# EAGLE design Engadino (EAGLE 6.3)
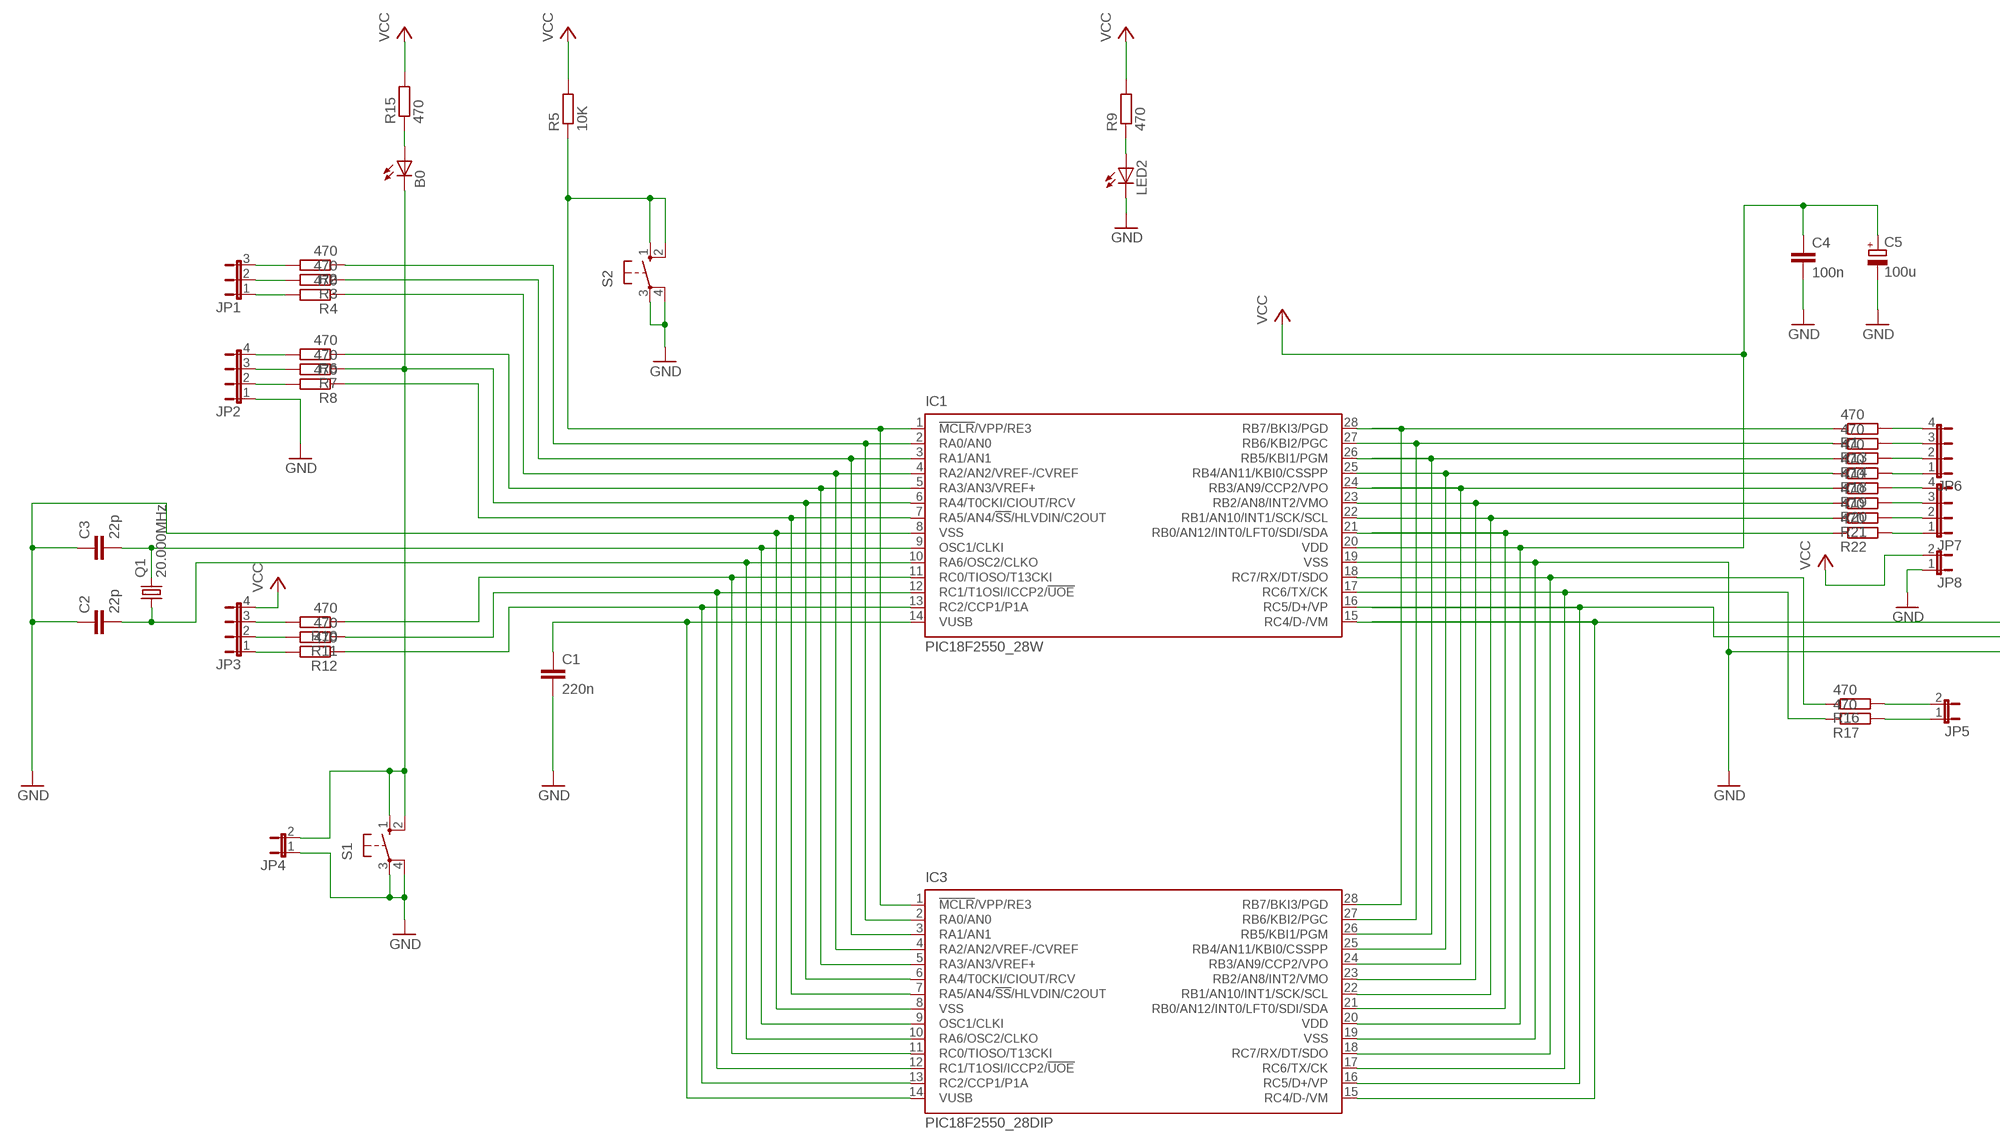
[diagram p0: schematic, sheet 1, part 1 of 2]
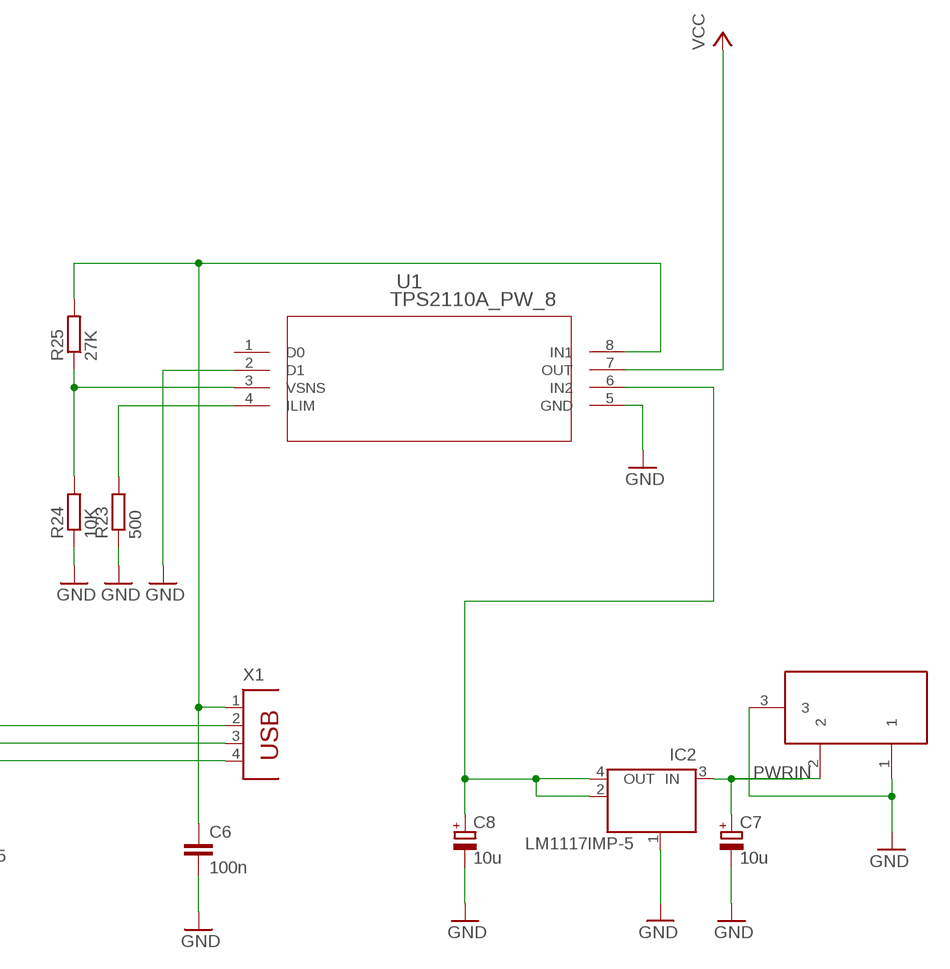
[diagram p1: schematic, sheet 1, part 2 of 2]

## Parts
B0  LEDCHIPLED_0805  [CHIPLED_0805]
C1  220n  C-EUC2012  [C2012]
C2  22p  C-EUC2012  [C2012]
C3  22p  C-EUC2012  [C2012]
C4  100n  C-EUC2012  [C2012]
C5  100u  CPOL-EU085CS-1AR  [085CS_1AR]
C6  100n  C-EUC2012  [C2012]
C7  10u  CPOL-EU085CS-1AR  [085CS_1AR]
C8  10u  CPOL-EU085CS-1AR  [085CS_1AR]
IC1  PIC18F2550_28W  [SO28W]
IC2  LM1117IMP-5  MC33269ST-3.3T3  [SOT223]
IC3  PIC18F2550_28DIP  [DIL28-3]
JP1  JP2E  [JP2]
JP2  JP4E  [JP4]
JP3  JP4E  [JP4]
JP4  JP1E  [JP1]
JP5  JP1E  [JP1]
JP6  JP4E  [JP4]
JP7  JP4E  [JP4]
JP8  JP1E  [JP1]
LED2  LEDCHIPLED_0805  [CHIPLED_0805]
Q1  20.000MHz  CRYSTALHC49S  [HC49/S]
R1  470  R-EU_R2012  [R2012]
R2  470  R-EU_R2012  [R2012]
R3  470  R-EU_R2012  [R2012]
R4  470  R-EU_R2012  [R2012]
R5  10K  R-EU_R2012  [R2012]
R6  470  R-EU_R2012  [R2012]
R7  470  R-EU_R2012  [R2012]
R8  470  R-EU_R2012  [R2012]
R9  470  R-EU_R2012  [R2012]
R10  470  R-EU_R2012  [R2012]
R11  470  R-EU_R2012  [R2012]
R12  470  R-EU_R2012  [R2012]
R13  470  R-EU_R2012  [R2012]
R14  470  R-EU_R2012  [R2012]
R15  470  R-EU_R2012  [R2012]
R16  470  R-EU_R2012  [R2012]
R17  470  R-EU_R2012  [R2012]
R18  470  R-EU_R2012  [R2012]
R19  470  R-EU_R2012  [R2012]
R20  470  R-EU_R2012  [R2012]
R21  470  R-EU_R2012  [R2012]
R22  470  R-EU_R2012  [R2012]
R23  500  R-EU_R2012  [R2012]
R24  10K  R-EU_R2012  [R2012]
R25  27K  R-EU_R2012  [R2012]
S1  10-XX  [B3F-10XX]
S2  10-XX  [B3F-10XX]
U1  TPS2110A_PW_8  [PW8]
X1  PN61729  [PN61729]
X2  DC21MMX  [DC-21MM]

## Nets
+5V: C8.+ IC2.2(OUT) IC2.4(OUT) U1.6(IN2)
GND: C1.2 C2.1 C3.1 C4.2 C5.- C6.2 C7.- C8.- IC1.8(VSS) IC1.19(VSS) IC2.1(GND/ADJ) IC3.8(VSS) IC3.19(VSS) JP2.1 JP4.1 JP8.1 LED2.C R23.1 R24.1 S1.3(P) S1.4(P1) S2.3(P) S2.4(P1) U1.2(D1) U1.5(GND) X1.4 X2.1 X2.3
GND2: IC1.21(RB0/AN12/INT0/LFT0/SDI/SDA) IC3.21(RB0/AN12/INT0/LFT0/SDI/SDA) R22.1
N$1: JP1.3 R2.2
N$2: IC1.15(RC4/D-/VM) IC3.15(RC4/D-/VM) X1.2
N$3: JP5.2 R16.2
N$4: JP5.1 R17.2
N$5: JP6.1 R18.2
N$9: JP1.2 R3.2
N$10: IC1.25(RB4/AN11/KBI0/CSSPP) IC3.25(RB4/AN11/KBI0/CSSPP) R18.1
N$11: JP7.4 R19.2
N$12: JP7.3 R20.2
N$13: JP6.4 R1.2
N$14: JP7.2 R21.2
N$15: IC1.24(RB3/AN9/CCP2/VPO) IC3.24(RB3/AN9/CCP2/VPO) R19.1
N$16: IC1.23(RB2/AN8/INT2/VMO) IC3.23(RB2/AN8/INT2/VMO) R20.1
N$17: JP1.1 R4.2
N$19: JP2.4 R6.2
N$20: JP2.3 R7.2
N$21: JP2.2 R8.2
N$23: JP3.3 R10.2
N$24: JP3.2 R11.2
N$25: JP3.1 R12.2
N$27: IC1.3(RA1/AN1) IC3.3(RA1/AN1) R3.1
N$33: JP6.3 R13.2
N$34: JP6.2 R14.2
N$35: LED2.A R9.1
N$38: IC1.22(RB1/AN10/INT1/SCK/SCL) IC3.22(RB1/AN10/INT1/SCK/SCL) R21.1
N$39: JP7.1 R22.2
N$41: IC1.18(RC7/RX/DT/SDO) IC3.18(RC7/RX/DT/SDO) R16.1
N$42: B0.A R15.1
N$43: IC1.28(RB7/BKI3/PGD) IC3.28(RB7/BKI3/PGD) R1.1
N$44: IC1.27(RB6/KBI2/PGC) IC3.27(RB6/KBI2/PGC) R13.1
N$45: IC1.17(RC6/TX/CK) IC3.17(RC6/TX/CK) R17.1
N$46: R23.2 U1.4(ILIM)
N$47: R24.2 R25.1 U1.3(VSNS)
N$48: IC1.26(RB5/KBI1/PGM) IC3.26(RB5/KBI1/PGM) R14.1
N$49: C6.1 R25.2 U1.8(IN1) X1.1
N$51: C1.1 IC1.14(VUSB) IC3.14(VUSB)
N$52: C3.2 IC1.9(OSC1/CLKI) IC3.9(OSC1/CLKI) Q1.2
N$53: C2.2 IC1.10(RA6/OSC2/CLKO) IC3.10(RA6/OSC2/CLKO) Q1.1
N$54: IC1.16(RC5/D+/VP) IC3.16(RC5/D+/VP) X1.3
N$55: IC1.2(RA0/AN0) IC3.2(RA0/AN0) R2.1
N$57: IC1.4(RA2/AN2/VREF-/CVREF) IC3.4(RA2/AN2/VREF-/CVREF) R4.1
N$58: IC1.5(RA3/AN3/VREF+) IC3.5(RA3/AN3/VREF+) R6.1
N$59: B0.C IC1.6(RA4/T0CKI/CIOUT/RCV) IC3.6(RA4/T0CKI/CIOUT/RCV) JP4.2 R7.1 S1.1(S) S1.2(S1)
N$60: IC1.7(RA5/AN4/!SS!/HLVDIN/C2OUT) IC3.7(RA5/AN4/!SS!/HLVDIN/C2OUT) R8.1
N$61: IC1.11(RC0/TIOSO/T13CKI) IC3.11(RC0/TIOSO/T13CKI) R10.1
N$62: IC1.12(RC1/T1OSI/ICCP2/!UOE) IC3.12(RC1/T1OSI/ICCP2/!UOE) R11.1
N$63: IC1.13(RC2/CCP1/P1A) IC3.13(RC2/CCP1/P1A) R12.1
N$64: IC1.1(!MCLR!/VPP/RE3) IC3.1(!MCLR!/VPP/RE3) R5.1 S2.1(S) S2.2(S1)
PWRIN: C7.+ IC2.3(IN) X2.2
VCC: C4.1 C5.+ IC1.20(VDD) IC3.20(VDD) JP3.4 JP8.2 R5.2 R9.2 R15.2 U1.7(OUT)
Unconnected: U1.1(D0)

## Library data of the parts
B0 LED2 = led:LED: LED
C1-C4 C6 = rcl:C-EU: CAPACITOR, European symbol
C5 C7 C8 = rcl:CPOL-EU: POLARIZED CAPACITOR, European symbol
IC1 IC3 = microchip:PIC18F2*_28: USB Microcontrollers with nanoWatt Technology High-Performance, Enhanced Flash, 28/40/44-Pin, Source: http://ww1.microchip.com/downloads/en/devicedoc/39632c.pdf
IC2 = linear:MC33269ST*: Adjustable Output Low Dropout Voltage Regulator 800 mA Source: http://www.onsemi.com/pub/Collateral/MC33269-D.PDF
JP1 = jumper:JP2E: JUMPER
JP2 JP3 JP6 JP7 = jumper:JP4E: JUMPER
JP4 JP5 JP8 = jumper:JP1E: JUMPER
Q1 = crystal:CRYSTAL: CRYSTAL
R1-R25 = rcl:R-EU_: RESISTOR, European symbol
S1 S2 = switch-omron:10-XX: OMRON SWITCH; MPN: B3F-1000; OC_FARNELL: 176432; OC_NEWARK: 36M3542
U1 = TPS2110A:TPS2110A_PW_8; DATASHEETURL: http://www.ti.com/lit/gpn/TPS2110A; DESCRIPTION: Autoswitching Power Mux; FAMILY_NAME: POWER MULTIPLEXER (MUX); GENERIC_PART_NUMBER: TPS2110A; INDUSTRY_STD_PKG_TYPE: TSSOP; MANUFACTURER: Texas Instruments; MANUFACTURER_PART_NUMBER: tps2110a_pw_8; PACKAGE_DESIGNATOR: PW; PIN_COUNT: 8; VENDOR: Texas Instruments
X1 = con-berg:PN61729: BERG USB connector
X2 = powersupply:DC21MM

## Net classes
0 default: width 0.203 mm, drill 0.406 mm, clearance 0.203 mm
2 gnd: width 0.305 mm, drill 0.711 mm, clearance 0.203 mm

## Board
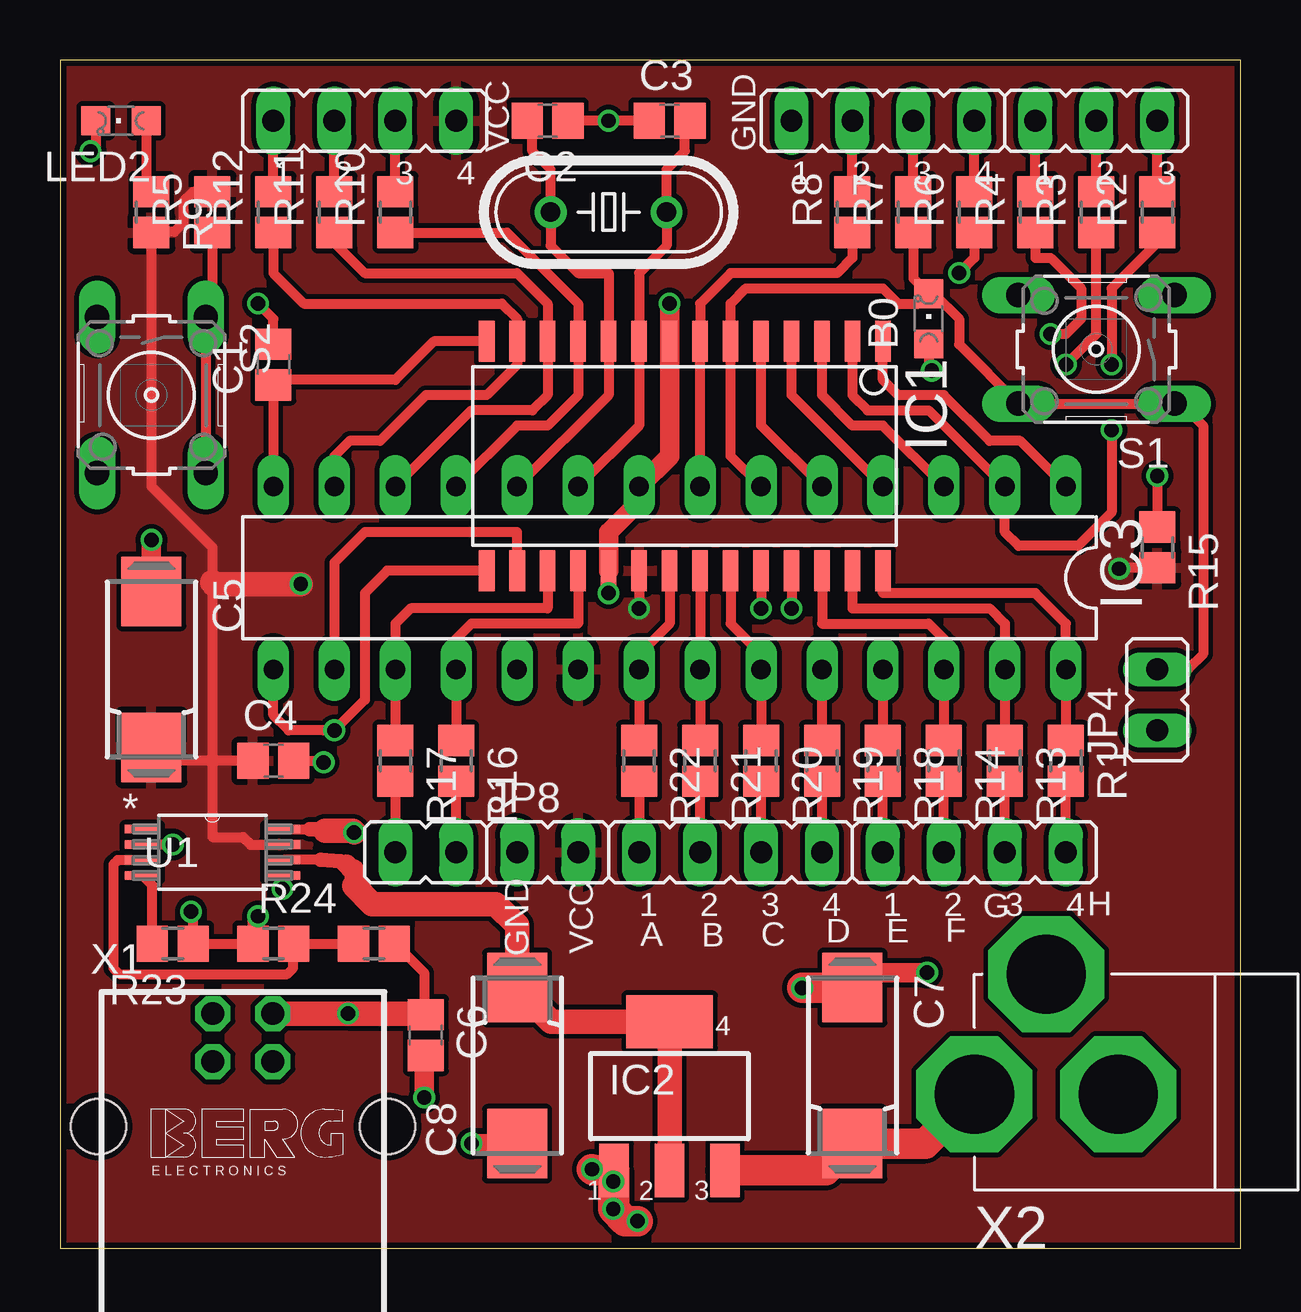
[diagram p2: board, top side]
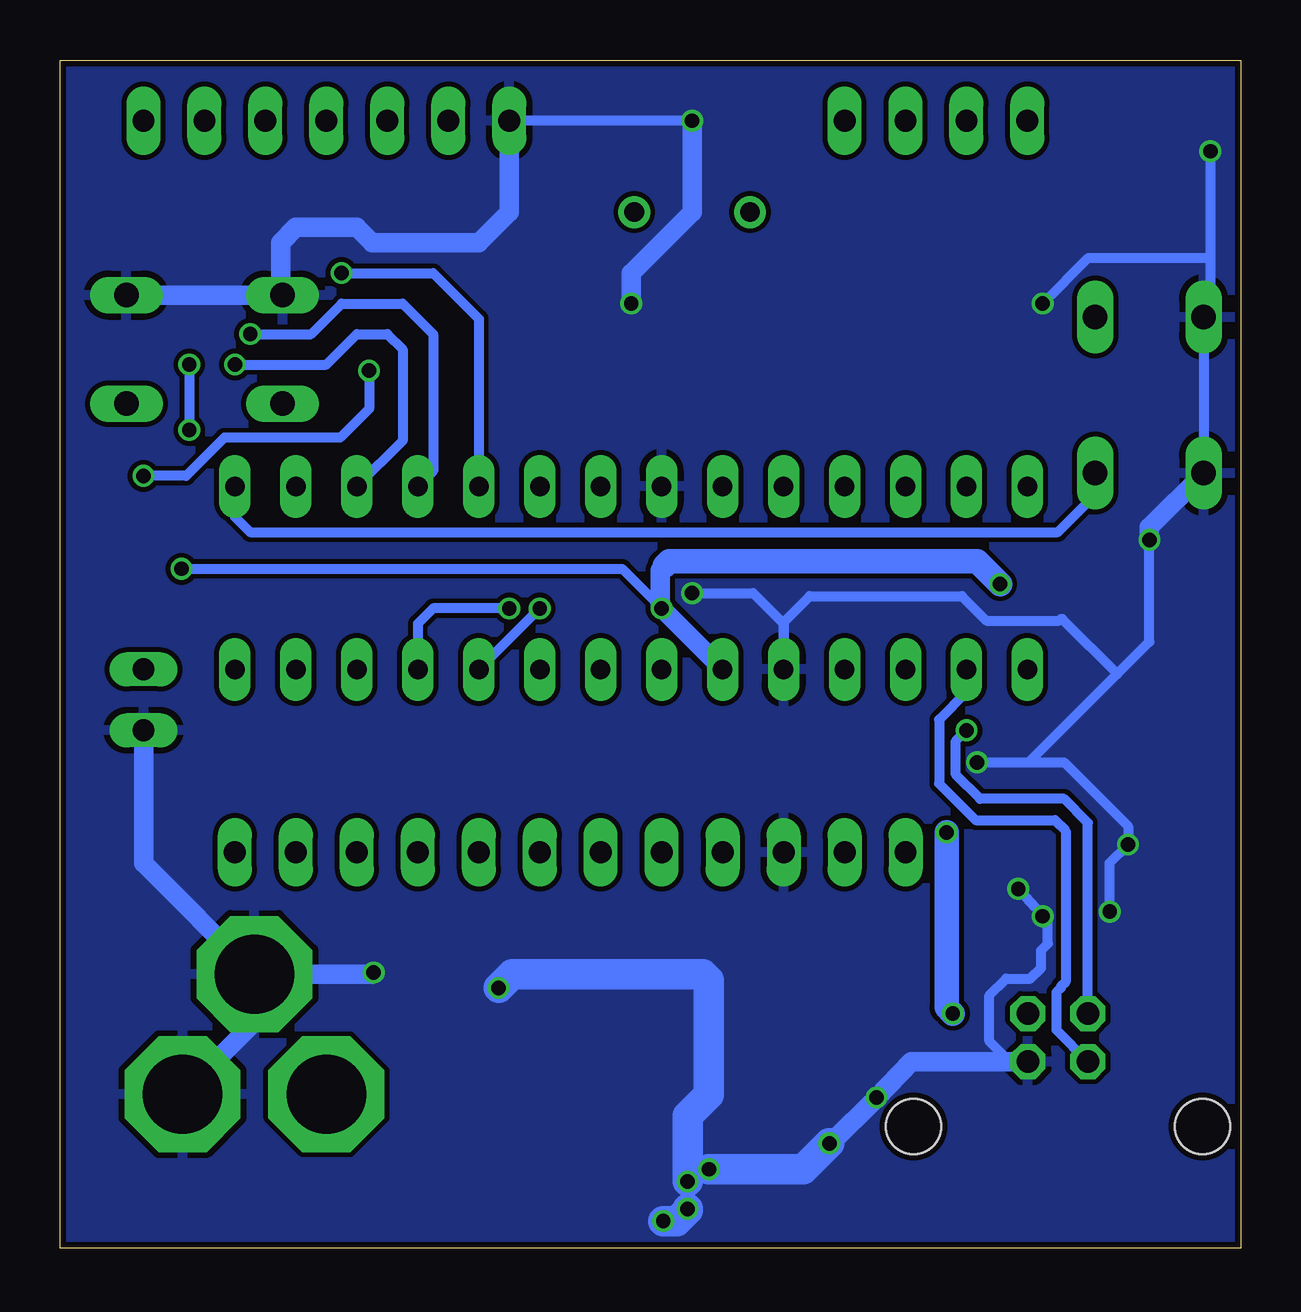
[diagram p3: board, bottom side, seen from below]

Size 49.2 x 49.52 mm. Coordinates in mm from the lower left corner, seen from the top.
Outline: 0,0 49.2,0 49.2,49.52 0,49.52 0,0
Copper layers (1*16): Top 0.035mm / dielectric 1.5mm / Bottom 0.035mm
Design rules "ITead_rule": minimum track width 6mil, minimum drill 12mil, track to track 6mil, track to pad 6mil, pad to pad 6mil, via to via 6mil, smd to smd 0mil, copper to edge 10mil, drill to drill 10mil, minimum pad ring 10mil, minimum via ring 6mil, stop-mask expansion 2mil, vias tented up to drill 100mil, thermal gap 10mil

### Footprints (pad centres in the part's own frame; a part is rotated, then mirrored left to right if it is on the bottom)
CHIPLED_0805 = smd 1.2 x 1.2: A 0,-1.05; C 0,1.05
C2012 = smd 1.3 x 1.5: 1 -0.85,0; 2 0.85,0
085CS_1AR = smd 2.9 x 2.5: + 3.25,0; - -3.25,0
SO28W = smd 0.65 x 1.7: 1 -7.62,-4.78; 2 -6.35,-4.78; 3 -5.08,-4.78; 4 -3.81,-4.78; 5 -2.54,-4.78; 6 -1.27,-4.78; 7 0,-4.78; 8 1.27,-4.78; 9 2.54,-4.78; 10 3.81,-4.78; 11 5.08,-4.78; 12 6.35,-4.78; 13 7.62,-4.78; 14 8.89,-4.78; 15 8.89,4.78; 16 7.62,4.78; 17 6.35,4.78; 18 5.08,4.78; 19 3.81,4.78; 20 2.54,4.78; 21 1.27,4.78; 22 0,4.78; 23 -1.27,4.78; 24 -2.54,4.78; 25 -3.81,4.78; 26 -5.08,4.78; 27 -6.35,4.78; 28 -7.62,4.78
SOT223 = smd 1.219 x 2.235: 1 -2.311,-3.099; 2 0,-3.099; 3 2.311,-3.099 | smd 3.6 x 2.2: 4 0,3.099
DIL28-3 = drill 0.813 long: 1 -16.51,-3.81; 2 -13.97,-3.81; 3 -11.43,-3.81; 4 -8.89,-3.81; 5 -6.35,-3.81; 6 -3.81,-3.81; 7 -1.27,-3.81; 8 1.27,-3.81; 9 3.81,-3.81; 10 6.35,-3.81; 11 8.89,-3.81; 12 11.43,-3.81; 13 13.97,-3.81; 14 16.51,-3.81; 15 16.51,3.81; 16 13.97,3.81; 17 11.43,3.81; 18 8.89,3.81; 19 6.35,3.81; 20 3.81,3.81; 21 1.27,3.81; 22 -1.27,3.81; 23 -3.81,3.81; 24 -6.35,3.81; 25 -8.89,3.81; 26 -11.43,3.81; 27 -13.97,3.81; 28 -16.51,3.81
JP2 = drill 0.914 long: 1 -2.54,0; 2 0,0; 3 2.54,0
JP4 = drill 0.914 long: 1 -3.81,0; 2 -1.27,0; 3 1.27,0; 4 3.81,0
JP1 = drill 0.914 long: 1 0,-1.27; 2 0,1.27
HC49/S = drill 0.813: 1 -2.413,0; 2 2.413,0
R2012 = smd 1.3 x 1.5: 1 -0.85,0; 2 0.85,0
B3F-10XX = drill 1.016 long: 1 -3.251,2.261; 2 3.251,2.261; 3 -3.251,-2.261; 4 3.251,-2.261
PW8 = smd 1.473 x 0.356: 1 -2.921,0.965; 2 -2.921,0.33; 3 -2.921,-0.33; 4 -2.921,-0.965; 5 2.921,-0.965; 6 2.921,-0.33; 7 2.921,0.33; 8 2.921,0.965
PN61729 = drill 0.95 octagon: 1 1.25,4.71; 2 -1.25,4.71; 3 -1.25,2.71; 4 1.25,2.71 | hole 2.3: -6.02,0; 6.02,0
DC-21MM = drill 3.302 pad 4.826 octagon: 1 -5.08,-3.353; 2 -0.076,-6.35; 3 -0.076,-0.356

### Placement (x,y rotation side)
B0  36.2,38.73 0 top
C1  8.89,36.83 90 top
C2  20.32,46.99 180 top
C3  25.4,46.99 0 top
C4  8.89,20.32 0 top
C5  3.81,24.13 270 top
C6  15.24,8.89 270 top
C7  33.02,7.62 270 top
C8  19.05,7.62 90 top
IC1  26.67,33.02 180 top
IC2  25.4,6.35 0 top
IC3  25.4,27.94 180 top
JP1  43.18,46.99 0 top
JP2  34.29,46.99 0 top
JP3  12.7,46.99 0 top
JP4  45.72,22.86 0 top
JP5  15.24,16.51 270 top
JP6  38.1,16.51 0 top
JP7  27.94,16.51 0 top
JP8  20.32,16.51 270 top
LED2  2.54,46.99 90 top
Q1  22.86,43.18 0 top
R1  41.91,20.32 270 top
R2  45.72,43.18 90 top
R3  43.18,43.18 90 top
R4  40.64,43.18 90 top
R5  6.35,43.18 90 top
R6  38.1,43.18 90 top
R7  35.56,43.18 90 top
R8  33.02,43.18 90 top
R9  3.81,43.18 270 top
R10  13.97,43.18 90 top
R11  11.43,43.18 90 top
R12  8.89,43.18 90 top
R13  39.37,20.32 270 top
R14  36.83,20.32 270 top
R15  45.72,29.21 270 top
R16  16.51,20.32 270 top
R17  13.97,20.32 270 top
R18  34.29,20.32 270 top
R19  31.75,20.32 270 top
R20  29.21,20.32 270 top
R21  26.67,20.32 270 top
R22  24.13,20.32 270 top
R23  4.7,12.7 180 top
R24  8.89,12.7 0 top
R25  13.08,12.7 0 top
S1  43.18,37.47 180 top
S2  3.81,35.56 270 top
U1  6.35,16.51 0 top
X1  7.62,5.08 0 top
X2  44.45,6.35 270 top

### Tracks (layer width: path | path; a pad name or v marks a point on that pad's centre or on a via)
+5V
  Top 0.406: 10.86,16.19 9.32,16.19 U1.6
  Top 0.61: 11.94,16 11.81,16 11.68,16.13 10.86,16.19
  Top 0.813: 12.26,15.11 12.26,15.81 12.13,15.81 11.94,16
  Top 1.016: IC2.2 IC2.4 20.47,9.45 C8.+ 19.05,13.46 18.16,14.35 13.02,14.35 12.26,15.11
GND  (via drill 0.6)
  Top 0.406: IC1.19 v22.86,27.3 | LED2.C 1.49,45.94 v1.27,45.72 | C1.2 8.89,38.73 v8.26,39.37 | C2.1 v22.86,46.99 C3.1 | C4.2 10.92,20.32 v10.99,20.26 | v8.26,13.84 8.04,13.82 R24.1 R23.1 5.55,13.82 v5.46,14.03 | v9.27,14.99 U1.5 | v4.7,16.83 3.44,16.83 U1.2
  Top 0.813: IC1.19 22.86,29.84 24.13,31.11 IC3.8 25.4,33.02 IC1.8 v25.4,39.37 | C5.- v3.81,29.53 | v36.13,11.49 33.64,11.49 C7.- | C8.- 17.16,4.37 v17.14,4.38 | v15.18,6.29 15.18,7.98 C6.2
  Top 1.27: v22.16,3.3 22.21,3.25 IC2.1 23.09,1.69 v23.05,1.65 | v24.07,1.14 23.56,1.14 v23.05,1.65 | v23.05,1.65 v23.05,2.79 | v30.92,10.86 33.01,10.86 C7.-
  Bottom 0.406: v22.86,27.3 20.32,27.3 19.05,26.04 IC3.19 19.05,26.1 17.97,27.18 11.62,27.18 10.6,26.16 7.56,26.16 7.49,26.23 7.43,26.23 5.14,23.94 | v1.27,45.72 1.27,41.27 | 1.27,41.27 1.27,39.09 S2.3 S2.4 | v8.26,39.37 6.35,41.27 1.27,41.27 | v22.86,46.99 JP2.1 | v10.99,20.26 8.83,20.26 | 8.83,20.26 5.14,23.94 | 5.14,23.94 3.81,25.27 v3.81,29.53 | v9.27,14.99 v8.26,13.84 8.04,13.82 R24.1 8.32,12.42 8.32,11.68 8.76,11.24 9.78,11.24 10.48,10.54 10.48,8.64 9.63,7.79 X1.4 | v5.46,14.03 5.46,16.07 v4.7,16.83 4.7,17.59 7.37,20.26 8.83,20.26
  Bottom 0.813: v25.4,39.37 25.4,40.64 22.86,43.18 v22.86,46.99 | JP2.1 30.48,43.18 31.75,41.91 36.2,41.91 36.83,42.55 39.37,42.55 40.01,41.91 40.01,39.8 S1.4 S1.3 | v3.81,29.53 3.81,30.05 S2.4 | JP4.1 45.72,16.05 X2.1 | X2.1 41.1,9.42 X2.3 | X2.1 36.2,11.43 v36.13,11.49 | v17.14,4.38 17.08,4.38 v15.18,6.29 13.74,7.79 X1.4
  Bottom 1.27: v22.16,3.3 18.22,3.3 v17.14,4.38 | v23.05,1.65 23.05,1.59 23.5,1.14 v24.07,1.14 | v23.05,2.79 23.05,5.52 22.16,6.41 22.16,11.18 22.42,11.43 30.35,11.43 v30.92,10.86
  pour Bottom: -1.27,49.53 49.53,49.53 49.53,-1.27 -1.27,-1.27
GND2
  Top 0.406: IC1.21 25.4,26.04 24.13,24.77 IC3.21 R22.1
N$1
  Top 0.406: R2.2 JP1.3
N$2  (via drill 0.6)
  Top 0.406: IC1.15 13.63,28.24 12.7,27.3 12.7,22.86 v11.43,21.59 10.99,21.59 9.53,21.59 8.89,22.23 IC3.15
  Bottom 0.406: X1.2 6.37,17.74 7.37,18.73 10.86,18.73 11.87,19.75 11.87,21.14 v11.43,21.59
N$3
  Top 0.406: JP5.2 R16.2
N$4
  Top 0.406: R17.2 JP5.1
N$5
  Top 0.406: JP6.1 R18.2
N$9
  Top 0.406: R3.2 JP1.2
N$10  (via drill 0.6)
  Top 0.406: IC1.25 v30.48,26.67 | IC3.25 R18.1
  Bottom 0.406: v30.48,26.67 33.66,26.67 34.29,26.04 IC3.25
N$11
  Top 0.406: JP7.4 R19.2
N$12
  Top 0.406: JP7.3 R20.2
N$13
  Top 0.406: JP6.4 R1.2
N$14
  Top 0.406: JP7.2 R21.2
N$15  (via drill 0.6)
  Top 0.406: IC1.24 v29.21,26.67 | R19.1 IC3.24
  Bottom 0.406: v29.21,26.67 IC3.24
N$16
  Top 0.406: IC1.23 27.94,26.04 29.21,24.77 IC3.23 R20.1
N$17
  Top 0.406: R4.2 JP1.1
N$19
  Top 0.406: R6.2 JP2.4
N$20
  Top 0.406: R7.2 JP2.3
N$21
  Top 0.406: R8.2 JP2.2
N$23
  Top 0.406: R10.2 JP3.3
N$24
  Top 0.406: R11.2 JP3.2
N$25
  Top 0.406: R12.2 JP3.1
N$27  (via drill 0.6)
  Top 0.406: IC3.3 34.29,34.29 33.02,34.29 31.75,35.56 IC1.3 | v41.91,36.83 43.18,38.1 R3.1
  Bottom 0.406: v41.91,36.83 38.1,36.83 36.83,38.1 35.56,38.1 34.92,37.47 34.92,33.66 IC3.3
N$33
  Top 0.406: JP6.3 R13.2
N$34
  Top 0.406: JP6.2 R14.2
N$35
  Top 0.406: LED2.A 3.59,44.25 R9.1
N$38
  Top 0.406: IC1.22 IC3.22 R21.1
N$39
  Top 0.406: R22.2 JP7.1
N$41
  Top 0.406: IC1.18 21.59,26.04 17.14,26.04 16.51,25.4 IC3.18 R16.1
N$42  (via drill 0.6)
  Top 0.406: B0.A 36.2,36.7 v36.32,36.58 | v45.72,32.19 R15.1
  Bottom 0.406: v36.32,36.58 36.32,34.99 37.53,33.78 42.35,33.78 43.94,32.19 v45.72,32.19
N$43
  Top 0.406: R1.1 IC3.28 41.91,26.04 40.64,27.3 34.29,27.3 IC1.28
N$44
  Top 0.406: IC1.27 33.02,26.67 38.73,26.67 39.37,26.04 IC3.27 R13.1
N$45
  Top 0.406: IC1.17 20.32,26.67 14.61,26.67 13.97,26.04 IC3.17 R17.1
N$46
  Top 0.406: R23.2 3.85,15.12 U1.4
N$47
  Top 0.406: R25.1 R24.2 9.72,12.68 9.72,11.68 9.46,11.43 2.48,11.43 2.22,11.68 2.22,16 2.4,16.18 U1.3
N$48
  Top 0.406: IC1.26 31.75,26.04 36.2,26.04 36.83,25.4 IC3.26 R14.1
N$49  (via drill 0.6)
  Top 0.406: R25.2 13.97,12.7 15.18,11.49 15.18,9.8 C6.1 | U1.8 10.4,17.48 10.41,17.46
  Top 0.61: 10.41,17.46 10.99,17.46 11.05,17.4
  Top 1.016: C6.1 15.24,9.79 v12,9.79 X1.1 | 11.05,17.4 12.19,17.4 v12.26,17.34
  Bottom 1.016: v12.26,17.34 12.26,10.04 v12,9.79
N$51
  Top 0.406: IC1.14 15.57,37.8 13.97,36.2 9.11,36.2 C1.1 IC3.14
N$52
  Top 0.406: IC3.9 24.13,34.29 IC1.9 24.13,40.64 25.27,41.78 Q1.2 25.27,44.96 26.04,45.72 26.04,46.77 C3.2
N$53
  Top 0.406: IC3.10 22.86,35.56 IC1.10 22.86,40.64 21.59,40.64 20.45,41.78 Q1.1 20.45,44.96 19.68,45.72 19.68,46.77 C2.2
N$54
  Top 0.406: IC1.16 19.05,29.84 12.7,29.84 11.43,28.57 IC3.16
  Bottom 0.406: IC3.16 11.43,23.18 12.57,22.04 12.57,19.37 11.05,17.84 7.75,17.84 7.3,17.4 7.3,11.11 7.49,10.92 7.49,10.86 7.68,10.67 7.68,9.1 X1.3
N$55  (via drill 0.6)
  Top 0.406: IC1.2 33.02,35.56 33.66,34.92 36.2,34.92 IC3.2 39.37,29.84 39.94,29.27 42.42,29.27 43.81,30.67 v43.81,34.1 | R2.1 45.72,41.91 43.81,40.01 v43.81,36.83
  Bottom 0.406: v43.81,36.83 v43.81,34.1
N$57  (via drill 0.6)
  Top 0.406: IC3.4 30.48,35.56 IC1.4 | R4.1 40.64,41.27 41.27,41.27 42.55,40.01 42.55,38.73 41.91,38.1 v41.27,38.1
  Bottom 0.406: v41.27,38.1 38.73,38.1 37.47,39.37 34.92,39.37 33.66,38.1 33.66,32.38 IC3.4
N$58  (via drill 0.6)
  Top 0.406: IC3.5 29.21,34.29 IC1.5 | R6.1 38.1,41.27 v37.47,40.64
  Bottom 0.406: v37.47,40.64 33.66,40.64 31.75,38.73 IC3.5
N$59
  Top 0.406: IC3.6 27.94,33.02 IC1.6 27.94,39.37 28.57,40.01 34.29,40.01 34.92,39.37 35.78,39.37 B0.C | R7.1 35.56,40.42 B0.C | B0.C 36.41,39.78 37.47,38.73 37.47,37.67 S1.2 S1.1 46.71,35.2 47.62,34.29 47.62,24.77 46.99,24.13 JP4.2
N$60
  Top 0.406: IC3.7 IC1.7 26.67,39.37 27.94,40.64 32.38,40.64 33.02,41.27 R8.1
N$61
  Top 0.406: IC3.11 19.05,34.29 20.32,34.29 21.59,35.56 IC1.11 21.59,39.37 18.63,42.33 R10.1
N$62
  Top 0.406: IC3.12 17.14,34.92 19.68,34.92 20.32,35.56 IC1.12 20.32,39.37 19.05,40.64 12.7,40.64 11.43,41.91 R11.1
N$63
  Top 0.406: IC3.13 11.43,33.02 12.06,33.66 13.34,33.66 15.24,35.56 17.78,35.56 19.05,36.83 IC1.13 19.05,38.73 18.41,39.37 10.16,39.37 8.89,40.64 R12.1
N$64
  Top 0.406: IC3.1 40.01,33.66 38.73,33.66 36.83,35.56 34.92,35.56 34.29,36.2 IC1.1 | R5.1 6.35,39.09 S2.1 S2.2
  Bottom 0.406: IC3.1 41.91,30.48 41.27,29.84 7.62,29.84 6.35,31.11 6.35,32.03 S2.2
PWRIN
  Top 1.27: IC2.3 31.9,3.25 C7.+ 36.04,4.37 X2.2
VCC  (via drill 0.6)
  Top 0.406: IC1.20 v24.13,26.67 | 6.35,20.32 6.35,27.75 6.35,29.21 3.81,31.75 R9.2 3.83,42.35 4.76,42.35 5.14,42.74 5.14,43.62 5.55,44.03 R5.2 | 6.35,20.32 4.37,20.32 C5.+ | C4.1 6.35,20.32 | 6.35,20.32 6.35,17.14 7.62,17.14 7.94,16.82 9.25,16.82 U1.7 | R15.2 44.17,28.36 v44.13,28.32
  Top 1.016: v10.03,27.69 6.41,27.69 6.35,27.75
  Bottom 0.406: v44.13,28.32 25.78,28.32 24.19,26.73 v24.13,26.67
  Bottom 0.813: v24.13,26.67 IC3.20 24.19,26.73 24.19,28.26 24,28.45
  Bottom 1.016: 24,28.45 23.81,28.64 10.99,28.64 v10.03,27.69
  pour Top: -1.27,50.8 50.8,50.8 50.8,-1.27 -1.27,-1.27

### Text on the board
tNames: VCC | GND | G | H | A | B | C | D | E | F | GND | VCC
